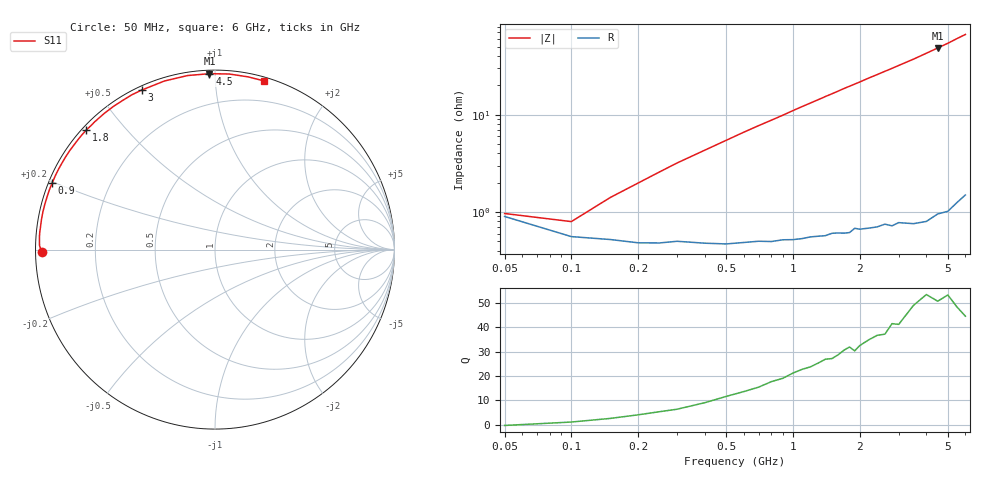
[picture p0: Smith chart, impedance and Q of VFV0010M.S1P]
! Infineon Technologies  Discrete & RF Semiconductors
! BBY 58-03
! Si Tuning Diode in SOD323
! VR =
! S-Parameters:  June  1999
# GHz  S  MA  R  50
!  f  S11
! GHz  MAG  ANG
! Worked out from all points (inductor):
!   34 points, 50 MHz to 6 GHz, reference 50 ohm
!   read as one part to ground: L = 1.61 nH near 200 MHz
!   highest Q = 53.4 at 4.5 GHz (marker M1), where L = 1.71 nH
!   S11 on the Smith chart (normalised r, x): 50 MHz: 0.02, -0.01; 900 MHz: 0.01, +0.20; 1.8 GHz: 0.01, +0.39; 3 GHz: 0.02, +0.64; 4.5 GHz: 0.02, +0.97; 6 GHz: 0.03, +1.33
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0.05  0.9647 -179.2
0.1  0.9779 178.7
0.15  0.9794 177.0
0.25  0.981 174.2
0.3  0.9803 172.8
0.4  0.9812 170.2
0.5  0.9816 167.6
0.6  0.9811 165.0
0.8  0.9809 160.1
0.9  0.9803 157.7
1  0.9804 155.2
1.1  0.9801 152.8
1.2  0.9795 150.5
1.4  0.9794 145.9
1.6  0.9786 141.5
1.8  0.9789 137.2
2  0.9778 133.2
2.2  0.978 129.1
2.4  0.9781 125.4
2.6  0.9774 121.7
2.8  0.979 118.2
3  0.9782 114.7
3.5  0.9807 106.7
4  0.9817 98.9
4.5  0.9805 91.8
5  0.9815 85.4
5.5  0.9799 79.1
6  0.9787 73.7
